ORGANIZATION_BLOCK OB 1
BEGIN
	CALL		FC 1
	CALL		FC 2
	CALL		FC 3
END_ORGANIZATION_BLOCK



FUNCTION FC 1: VOID
  VAR_INPUT
    INPUT_WORD : WORD
  END_VAR
BEGIN
	U		E 0.0
	=		A 0.0
END_FUNCTION



FUNCTION FC 2: VOID
TITLE = Shift register
BEGIN
	UN		T 10
	=		M 0.0
	L		S5T#200MS
	SV		T 10

	L		MD 4
	L		1
	==D
	S		M 0.1
	RRD		1
	==D
	R		M 0.1

	L		MD 4
	UD		L#-1
	L		1
	SPZ		_001
	TAK
	U		M 0.0
	SPBN		_001
	U		M 0.1
	SPBN		_000
	RLD		2
_000:	RRD		1
_001:	T		MD 4

	L		MD 4
	T		AD 4
	TAD
	T		AD 8
END_FUNCTION



FUNCTION FC 3: VOID
TITLE = DB usage example
BEGIN
	AUF		DB 1
	L		DBD 2
END_FUNCTION



DATA_BLOCK DB 1
TITLE = This is DB 1
STRUCT
	VAR1 : INT		// DBW0: VAR1 => 16 bit signed int
	VAR2 : DWORD	// DBD2: VAR2 => 32 bit unsigned dword
	VAR3 : WORD		// DBW6: VAR3 => 16 bit unsigned word
END_STRUCT
BEGIN
	VAR1 := 1337
	VAR2 := DW#16#DEADBEEF
	VAR3 := B#(1, 2)
END_DATA_BLOCK
